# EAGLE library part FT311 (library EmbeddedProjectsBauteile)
FTDI USB ANDROID Host IC
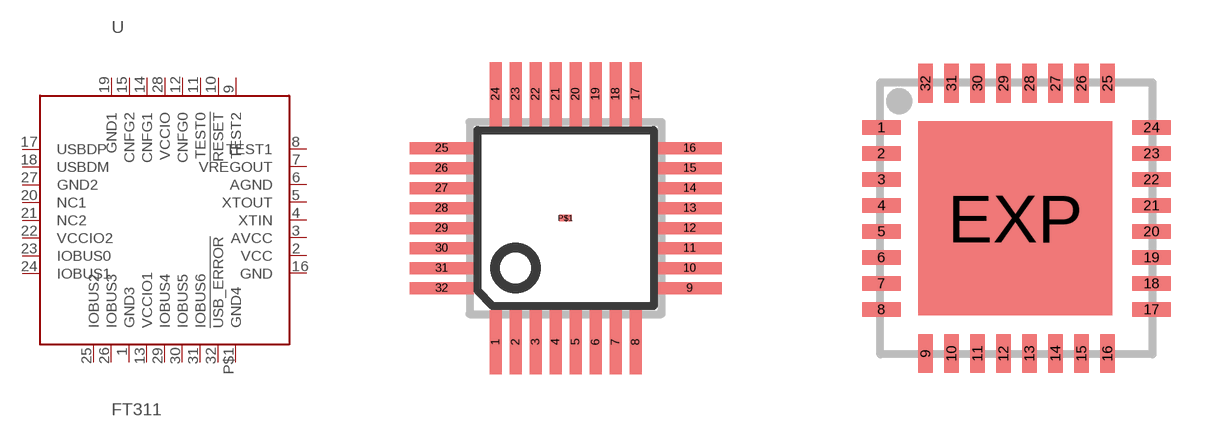
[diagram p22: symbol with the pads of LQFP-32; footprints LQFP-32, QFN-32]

Designator prefix -

## FT311LQFP-32 (EP: 400840)  [LQFP-32]
1  GND3  pwr
2  VCC  pwr
3  AVCC  pwr
4  XTIN  in
5  XTOUT  out
6  AGND  pwr
7  VREGOUT  out
8  TEST1  in
9  TEST2  in
10  !RESET  in
11  TEST0  in
12  CNFG0
13  VCCIO1  pwr
14  CNFG1
15  CNFG2
16  GND  pwr
17  USBDP
18  USBDM
19  GND1  pwr
20  NC1  nc
21  NC2  nc
22  VCCIO2  pwr
23  IOBUS0
24  IOBUS1
25  IOBUS2
26  IOBUS3
27  GND2  pwr
28  VCCIO  pwr
29  IOBUS4
30  IOBUS5
31  IOBUS6
32  !USB_ERROR
P$1  GND4  pwr

## FT311TQFN-32  [QFN-32]
1  GND4  pwr
2  VCC  pwr
3  AVCC  pwr
4  XTIN  in
5  XTOUT  out
6  AGND  pwr
7  VREGOUT  out
8  TEST1  in
9  TEST2  in
10  !RESET  in
11  TEST0  in
12  CNFG0
13  VCCIO  pwr
14  CNFG1
15  CNFG2
16  GND1  pwr
17  USBDP
18  USBDM
19  GND2  pwr
20  NC1  nc
21  NC2  nc
22  VCCIO1  pwr
23  IOBUS0
24  IOBUS1
25  IOBUS2
26  IOBUS3
27  GND3  pwr
28  VCCIO2  pwr
29  IOBUS4
30  IOBUS5
31  IOBUS6
32  !USB_ERROR
EXP  GND  pwr

## Footprint LQFP-32 (pad centres in mm)
smd 0.3 x 1.6: 1 -1.75,-3.1; 2 -1.25,-3.1; 3 -0.75,-3.1; 4 -0.25,-3.1; 5 0.25,-3.1; 6 0.75,-3.1; 7 1.25,-3.1; 8 1.75,-3.1; 17 1.75,3.1; 18 1.25,3.1; 19 0.75,3.1; 20 0.25,3.1; 21 -0.25,3.1; 22 -0.75,3.1; 23 -1.25,3.1; 24 -1.75,3.1
smd 1.6 x 0.3: 9 3.1,-1.75; 10 3.1,-1.25; 11 3.1,-0.75; 12 3.1,-0.25; 13 3.1,0.25; 14 3.1,0.75; 15 3.1,1.25; 16 3.1,1.75; 25 -3.1,1.75; 26 -3.1,1.25; 27 -3.1,0.75; 28 -3.1,0.25; 29 -3.1,-0.25; 30 -3.1,-0.75; 31 -3.1,-1.25; 32 -3.1,-1.75
smd 0.305 x 0.152: P$1 0,0

## Footprint QFN-32 (pad centres in mm)
smd 0.965 x 0.366: 1 -3.418,2.295; 2 -3.418,1.645; 3 -3.418,0.995; 4 -3.418,0.345; 5 -3.418,-0.305; 6 -3.418,-0.955; 7 -3.418,-1.605; 8 -3.418,-2.255; 17 3.338,-2.255; 18 3.338,-1.605; 19 3.338,-0.955; 20 3.338,-0.305; 21 3.338,0.345; 22 3.338,0.995; 23 3.338,1.645; 24 3.338,2.295
smd 0.366 x 0.965: 9 -2.315,-3.358; 10 -1.665,-3.358; 11 -1.015,-3.358; 12 -0.365,-3.358; 13 0.285,-3.358; 14 0.935,-3.358; 15 1.585,-3.358; 16 2.235,-3.358; 25 2.235,3.398; 26 1.585,3.398; 27 0.935,3.398; 28 0.285,3.398; 29 -0.365,3.398; 30 -1.015,3.398; 31 -1.665,3.398; 32 -2.315,3.398
smd 4.851 x 4.851: EXP -0.07,0.02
